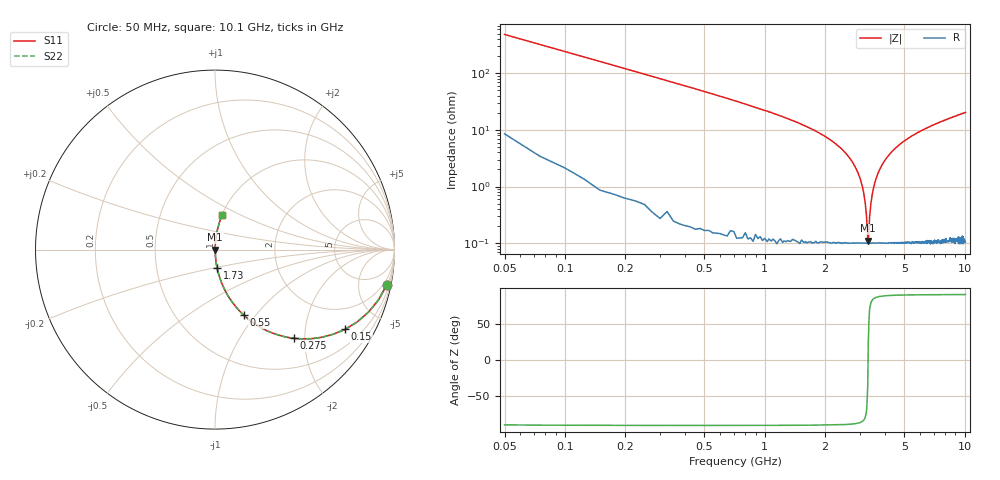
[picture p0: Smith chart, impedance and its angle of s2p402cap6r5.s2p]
! AVX Thin Film Operation		Date: April 2003
! Description: Accu-P® Series, Thin Film, SMD, RF Capacitor
! Part Number: 04025J6R5BBS
! 50 MHz  -  10.05 GHz
! Serial Measurements
# hz S db R 50
!	S11		S21		S12		S22
!	dB	Phase	dB	Phase	dB	Phase	dB	Phase
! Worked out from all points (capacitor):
!   400 points, 50 MHz to 10.1 GHz, reference 50 ohm
!   read as one part in series: C = 6.5 pF near 100 MHz
!   lowest |Z| = 110 mohm at 3.3 GHz (marker M1)
!   series resonance near 3.292 GHz, so ESL is about 360 pH
!   S11 on the Smith chart (normalised r, x): 50 MHz: 1.17, -9.79; 150 MHz: 1.02, -3.25; 275 MHz: 1.01, -1.77; 550 MHz: 1.00, -0.87; 1.73 GHz: 1.00, -0.21; 10.1 GHz: 1.00, +0.41
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5e7  -0.21 -11.5  -14.00 77.5  -14.00 77.5  -0.21 -11.5
1e8  -0.70 -22.2  -8.47 67.3  -8.47 67.3  -0.70 -22.2
1.5e8  -1.41 -31.5  -5.65 58.2  -5.65 58.2  -1.41 -31.5
2.75e8  -3.60 -48.4  -2.53 41.4  -2.53 41.4  -3.60 -48.4
5.5e8  -8.03 -66.4  -0.76 23.4  -0.76 23.4  -8.03 -66.4
1.73e9  -19.80 -83.6  -0.05 5.9  -0.05 5.9  -19.80 -83.6
2.43e9  -26.70 -86.1  -0.02 2.6  -0.02 2.6  -26.70 -86.1
2.93e9  -35.10 -85.7  -0.01 1.0  -0.01 1.0  -35.10 -85.7
3.08e9  -39.90 -83.8  -0.01 0.6  -0.01 0.6  -39.90 -83.8
3.18e9  -45.40 -79.0  -0.01 0.3  -0.01 0.3  -45.40 -79.0
3.23e9  -50.10 -71.3  -0.01 0.2  -0.01 0.2  -50.10 -71.3
3.28e9  -58.30 -34.4  -0.01 0.0  -0.01 0.0  -58.30 -34.4
3.3e9  -59.20 24.0  -0.01 -0.0  -0.01 -0.0  -59.20 24.0
3.35e9  -50.90 69.4  -0.01 -0.2  -0.01 -0.2  -50.90 69.4
3.4e9  -46.00 78.2  -0.01 -0.3  -0.01 -0.3  -46.00 78.2
3.6e9  -37.40 85.0  -0.01 -0.8  -0.01 -0.8  -37.40 85.0
3.9e9  -31.90 86.3  -0.01 -1.5  -0.01 -1.5  -31.90 86.3
4.35e9  -27.50 86.2  -0.02 -2.4  -0.02 -2.4  -27.50 86.2
5.08e9  -23.60 85.3  -0.03 -3.8  -0.03 -3.8  -23.60 85.3
6.75e9  -18.70 82.9  -0.07 -6.6  -0.07 -6.6  -18.70 82.9
8.43e9  -16.00 80.4  -0.12 -9.2  -0.12 -9.2  -16.00 80.4
1.01e10  -14.00 78.2  -0.18 -11.5  -0.18 -11.5  -14.00 78.2
